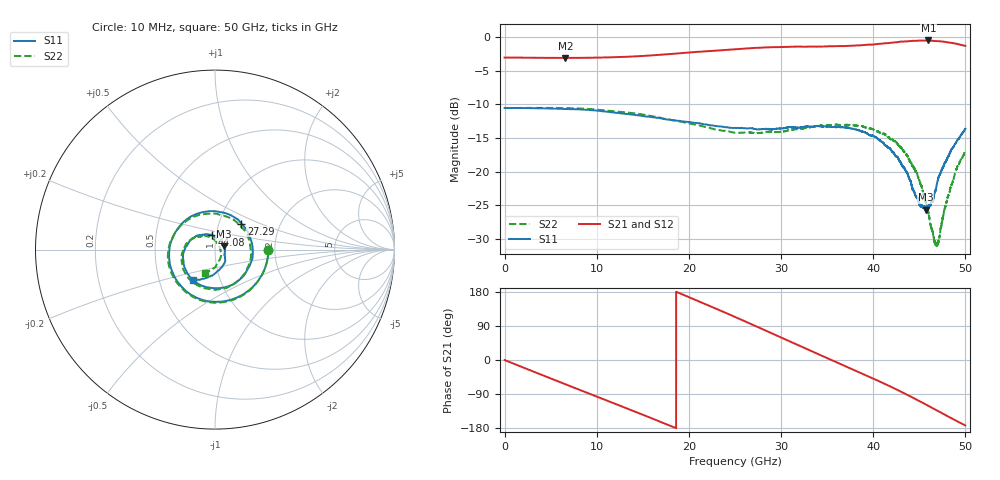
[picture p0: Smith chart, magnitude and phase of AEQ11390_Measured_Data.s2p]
!The following data was pulled from an Agilent PNA
!This sNp file was generated from the data in the RF Test software
!NOTE:  Smoothing/Math/Corrections applied on any given trace ARE included in the data saved here
# MHz S dB R 50
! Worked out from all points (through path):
!   12801 points, 10 MHz to 50 GHz, reference 50 ohm
!   highest |S21| = -0.53 dB at 45.98 GHz (marker M1); lowest = -3.1 dB at 6.606 GHz (marker M2)
!   group delay of S21, straight-line fit = 29.2 ps
!   lowest |S11| = -25.6 dB at 45.71 GHz (marker M3), VSWR 1.11, Z = 55.2 + j1.93 ohm
!   |S11| at or under -10 dB: start of sweep to end of sweep
!   |S22| runs from -31.0 to -10.5 dB; largest |S21 - S12| = 0.0028
!   S11 on the Smith chart (normalised r, x): 10 MHz: 1.85, -0.00; 27.29 GHz: 1.28, +0.39; 44.08 GHz: 0.95, +0.16; 50 GHz: 0.74, -0.26
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10  -10.54 -0.2  -3.07 -0.1  -3.06 -0.1  -10.54 -0.1
3064.077  -10.57 -38.7  -3.09 -29.9  -3.09 -29.9  -10.53 -38.9
6606.337  -10.68 -81.3  -3.12 -64.0  -3.11 -64.1  -10.55 -81.6
8344.271  -10.76 -101.1  -3.11 -80.7  -3.10 -80.7  -10.63 -101.3
12308.32  -11.28 -143.4  -3.00 -118.6  -3.00 -118.6  -11.08 -143.3
16674.63  -11.99 173.1  -2.67 -160.8  -2.67 -160.9  -11.92 172.0
20748.04  -12.76 131.2  -2.23 158.2  -2.23 158.1  -13.04 130.6
25005  -13.49 78.9  -1.82 113.7  -1.82 113.6  -14.21 78.5
27289.7  -13.69 44.5  -1.62 88.9  -1.62 88.8  -14.27 45.6
30171.94  -13.56 -0.2  -1.50 57.5  -1.50 57.4  -14.03 0.9
33339.27  -13.34 -54.3  -1.43 22.8  -1.43 22.8  -13.35 -49.1
35358.4  -13.37 -89.0  -1.38 1.1  -1.38 1.1  -13.12 -80.7
37455.63  -13.51 -123.1  -1.32 -21.3  -1.32 -21.4  -13.10 -111.9
39326.36  -14.32 -154.4  -1.17 -41.6  -1.17 -41.7  -13.49 -139.9
41669.64  -16.42 164.2  -0.91 -67.8  -0.92 -67.9  -14.92 -176.2
44075.4  -21.47 102.5  -0.61 -96.6  -0.61 -96.7  -18.66 141.9
45711.8  -25.60 19.4  -0.54 -117.4  -0.54 -117.6  -24.47 98.1
45981.27  -25.10 -3.7  -0.53 -121.0  -0.53 -121.1  -26.00 87.2
46645.2  -23.18 -36.6  -0.61 -129.7  -0.61 -129.8  -30.41 40.4
46988.88  -21.38 -48.9  -0.64 -134.1  -0.64 -134.2  -30.83 2.7
48265.97  -17.35 -91.3  -0.85 -150.8  -0.86 -150.9  -23.13 -72.7
50000  -13.62 -125.7  -1.33 -172.8  -1.34 -172.9  -16.84 -112.3
